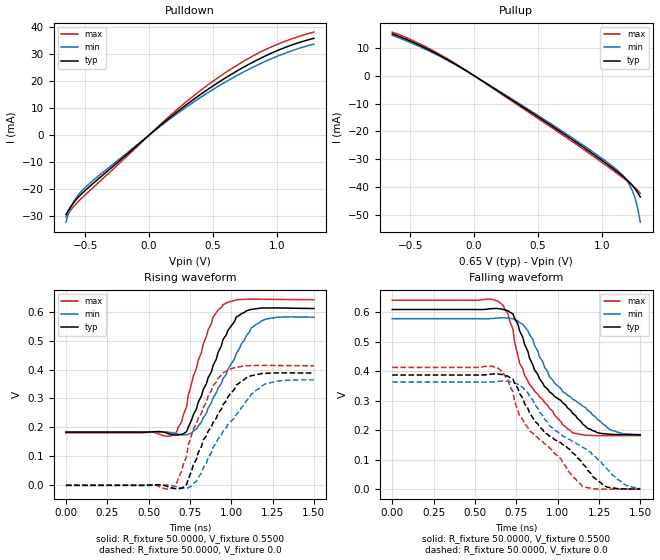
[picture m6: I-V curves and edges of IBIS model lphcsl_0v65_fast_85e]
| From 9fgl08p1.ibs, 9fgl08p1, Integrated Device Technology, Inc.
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[Model]   lphcsl_0v65_fast_85e
Model_type Output
Polarity   Inverting
Enable   Active-High
Vmeas =  0.4000V
Cref =   2.0000pF
Rref =   0.0
Vref =   0.4000V
C_comp   1.1000pF   1.0000pF   1.2000pF
[Temperature Range]   25.0000   85.0000   -40.0000
[Voltage Range]   0.6500V   0.6200V   0.6800V
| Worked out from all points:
|   slope of the pulldown table from 0 to 0.098 V, typ, clamps not added: 24.6 ohm
|   slope of the pullup table from 0 to 0.098 V, typ, clamps not added: 34 ohm
|   rising waveform, R_fixture 50.0000, V_fixture 0.5500: 20-80 % time 181ps typ, 222ps min, 141ps max; typ from 0.184 V to 0.611 V
|   rising waveform, R_fixture 50.0000, V_fixture 0.0: 20-80 % time 209ps typ, 245ps min, 165ps max; typ from 0 V to 0.388 V
|   falling waveform, R_fixture 50.0000, V_fixture 0.5500: 20-80 % time 293ps typ, 338ps min, 226ps max; typ from 0.61 V to 0.184 V
|   falling waveform, R_fixture 50.0000, V_fixture 0.0: 20-80 % time 379ps typ, 434ps min, 312ps max; typ from 0.387 V to 0 V
[Pulldown]
|Voltage   I(typ)   I(min)   I(max)
-650mV    -29.53mA   -32.32mA   -30.49mA
-630mV    -27.88mA   -29.08mA   -28.98mA
-590mV    -25.09mA   -24.79mA   -26.48mA
-550mV    -22.86mA   -21.99mA   -24.47mA
-510mV    -20.99mA   -19.89mA   -22.65mA
-370mV    -15.18mA   -14.16mA   -16.53mA
10mV      415.6uA    382.9uA    460.3uA
230mV     9.045mA    8.358mA    9.971mA
510mV     18.6mA     17.25mA    20.36mA
770mV     26.03mA    24.22mA    28.28mA
1.01V     31.54mA    29.44mA    33.86mA
1.29V     35.98mA    33.84mA    38.29mA
[Pullup]
|Voltage   I(typ)   I(min)   I(max)
-640mV    15.06mA    14.49mA    15.68mA
-520mV    12.87mA    12.35mA    13.49mA
-360mV    9.457mA    9.049mA    9.963mA
-60mV     1.732mA    1.649mA    1.841mA
600mV     -17.81mA   -17.25mA   -18.45mA
1.06V     -32.46mA   -31.73mA   -33.16mA
1.16V     -35.99mA   -35.72mA   -36.56mA
1.22V     -38.54mA   -39.59mA   -38.7mA
1.24V     -39.57mA   -41.53mA   -39.46mA
1.26V     -40.75mA   -44.1mA    -40.29mA
1.28V     -42.07mA   -47.64mA   -41.21mA
1.3V      -43.57mA   -52.66mA   -42.27mA
[Ramp]
| variable   typ   min   max
dV/dt_r  0.2327/0.2095n   0.2185/0.2437n   0.2478/0.1776n
dV/dt_f  0.2587/0.2708n   0.2393/0.3142n   0.2797/0.2305n
R_load = 50.0000
[Rising Waveform]
R_fixture= 50.0000
V_fixture= 0.5500
V_fixture_min= 0.5200
V_fixture_max= 0.5800
|time   V(typ)   V(min)   V(max)
0s        184mV      183.2mV    181.4mV
620ps     178.2mV    183.7mV    169.7mV
670ps     173.4mV    178.4mV    184.7mV
710ps     178.2mV    174.6mV    243.8mV
790ps     264.8mV    194.6mV    404mV
860ps     371.7mV    266.9mV    537.2mV
950ps     503.7mV    368.2mV    623.5mV
1.03ns    581.2mV    455.2mV    640.7mV
1.15ns    610mV      555.9mV    643.2mV
1.5ns     610.6mV    580.7mV    641.1mV
[Rising Waveform]
R_fixture= 50.0000
V_fixture= 0.0
V_fixture_min= 0.0
V_fixture_max= 0.0
|time   V(typ)   V(min)   V(max)
0s        0V         0V         0V
620ps     -5.715mV   709uV      -13.29mV
700ps     -9.925mV   -8.803mV   48.91mV
730ps     3.232mV    -10.2mV    100.5mV
770ps     70mV       5.855mV    193.5mV
890ps     217.3mV    131.5mV    344.4mV
950ps     278.4mV    186.5mV    388.4mV
1.06ns    359.7mV    267.6mV    410.8mV
1.2ns     386.3mV    348.4mV    414.1mV
1.5ns     387.8mV    364.2mV    413mV
[Falling Waveform]
R_fixture= 50.0000
V_fixture= 0.5500
V_fixture_min= 0.5200
V_fixture_max= 0.5800
|time   V(typ)   V(min)   V(max)
0s        609.5mV    578.3mV    640.9mV
590ps     611.7mV    578.5mV    644.9mV
700ps     604.9mV    580.7mV    595.3mV
730ps     594.3mV    577.9mV    542.1mV
770ps     537.2mV    565.6mV    427.3mV
800ps     490.8mV    551.2mV    386.4mV
920ps     348.1mV    414.9mV    294mV
1.03ns    293.2mV    330.6mV    218mV
1.24ns    191.1mV    236.3mV    181mV
1.5ns     184.1mV    184.4mV    181.3mV
[Falling Waveform]
R_fixture= 50.0000
V_fixture= 0.0
V_fixture_min= 0.0
V_fixture_max= 0.0
|time   V(typ)   V(min)   V(max)
0s        387mV      363mV      412.8mV
590ps     389.3mV    363.2mV    417.2mV
700ps     382.8mV    366mV      370.6mV
770ps     324.3mV    350.8mV    248.2mV
830ps     258.1mV    315mV      196.9mV
950ps     179.5mV    214.4mV    139.8mV
1.15ns    86.23mV    141.6mV    7.819mV
1.3ns     6.047mV    66.36mV    -629.5uV
1.41ns    292.5uV    13.48mV    -317.3uV
1.5ns     -140.4uV   1.344mV    -113.4uV
